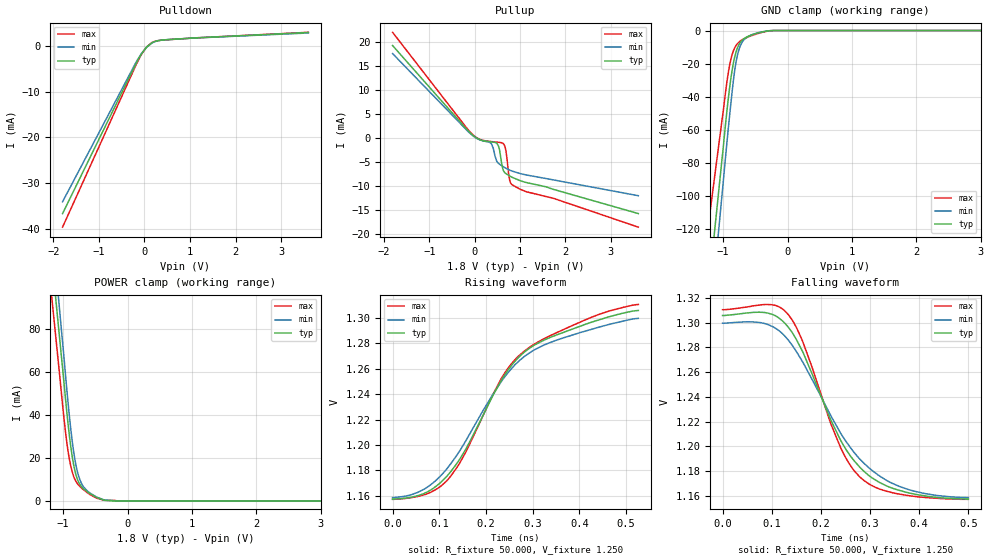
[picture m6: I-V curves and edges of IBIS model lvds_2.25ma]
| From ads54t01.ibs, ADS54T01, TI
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[Model]   lvds_2.25ma
Model_type 3-state
Vref=1.250E+00
Rref=5.000E+01
Cref=0.000E+00
Vmeas=1.250E+00
C_comp   7.860E-13   7.790E-13   7.930E-13
[Voltage Range]   1.800E+00   1.650E+00   1.950E+00
[POWER Clamp Reference]   1.800E+00   1.650E+00   1.950E+00
[GND Clamp Reference]   0.000E+00   0.000E+00   0.000E+00
[Pullup Reference]   1.800E+00   1.650E+00   1.950E+00
[Pulldown Reference]   0.000E+00   0.000E+00   0.000E+00
[Temperature Range]   25   85   -40
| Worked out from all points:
|   slope of the pulldown table from 0 to 0.27 V, typ, clamps not added: 137 ohm
|   slope of the pullup table from 0 to 0.27 V, typ, clamps not added: 279 ohm
|   GND clamp passes 1 mA (typ) near -0.41 V on its own axis
|   POWER clamp passes 1 mA (typ) near -0.41 V on its own axis
|   rising waveform, R_fixture 50.000, V_fixture 1.250: 20-80 % time 153ps typ, 161ps min, 159ps max; typ from 1.16 V to 1.31 V
|   falling waveform, R_fixture 50.000, V_fixture 1.250: 20-80 % time 107ps typ, 128ps min, 87.4ps max; typ from 1.31 V to 1.16 V
[GND Clamp]
-1.8V     -374.4mA   -423.5mA   -288.4mA
-1.02V    -78.69mA   -100.5mA   -54.92mA
-920mV    -41.17mA   -59.34mA   -25.51mA
-860mV    -23.88mA   -36.88mA   -14.48mA
-820mV    -15.94mA   -23.97mA   -10.43mA
-780mV    -10.76mA   -15.27mA   -8.038mA
-740mV    -7.589mA   -9.923mA   -6.562mA
-700mV    -5.657mA   -6.755mA   -5.499mA
-640mV    -4.069mA   -4.329mA   -4.359mA
-460mV    -1.489mA   -1.354mA   -1.806mA
-220mV    -4.201uA   -14.01uA   -11.29uA
3.6V      0A         0A         0A
[Power Clamp]
-1.8V     302.8mA    334.3mA    279.3mA
-1.76V    290.6mA    320.1mA    266.6mA
-1.06V    77.25mA    90.47mA    60.21mA
-940mV    40.5mA     50.88mA    26.54mA
-880mV    24.97mA    33.1mA     16.1mA
-820mV    14.43mA    19.78mA    10.24mA
-780mV    10.23mA    13.83mA    8.195mA
-720mV    6.913mA    8.542mA    6.262mA
-580mV    3.451mA    3.702mA    2.982mA
-360mV    441.4uA    538.8uA    356.5uA
-140mV    0A         9.789uA    18.55uA
3.6V      0A         0A         0A
[Pullup]
-1.81V    19.33mA    17.65mA    22.08mA
-30mV     540.2uA    453.4uA    652.3uA
370mV     -758.1uA   -1.136mA   -694.7uA
490mV     -1.048mA   -4.86mA    -804.7uA
530mV     -1.71mA    -5.276mA   -841.6uA
610mV     -5.976mA   -5.803mA   -982.6uA
650mV     -7.009mA   -6.039mA   -1.331mA
690mV     -7.357mA   -6.253mA   -2.621mA
770mV     -7.838mA   -6.622mA   -8.652mA
830mV     -8.153mA   -6.853mA   -9.716mA
1.15V     -9.25mA    -7.667mA   -11.17mA
3.61V     -15.7mA    -11.97mA   -18.53mA
[Pulldown]
-1.8V     -36.72mA   -34.13mA   -39.7mA
-180mV    -3.677mA   -3.428mA   -3.97mA
-80mV     -1.889mA   -1.783mA   -2.015mA
40mV      -299.8uA   -311.3uA   -270.9uA
160mV     724.9uA    669.1uA    793.7uA
320mV     1.262mA    1.247mA    1.257mA
520mV     1.453mA    1.46mA     1.421mA
3.6V      3.006mA    2.903mA    3.048mA
[Rising Waveform]
R_fixture = 50.000
V_fixture = 1.250
V_fixture_min = 1.250
V_fixture_max = 1.250
|  time   V(typ)   V(min)   V(max)
0s        1.157V     1.159V     1.157V
70ps      1.162V     1.166V     1.161V
120ps     1.177V     1.183V     1.173V
156ps     1.196V     1.203V     1.194V
234ps     1.252V     1.251V     1.253V
260ps     1.265V     1.262V     1.266V
288ps     1.275V     1.271V     1.276V
338ps     1.285V     1.281V     1.286V
428ps     1.297V     1.291V     1.301V
526ps     1.306V     1.3V       1.31V
[Falling Waveform]
R_fixture = 50.000
V_fixture = 1.250
V_fixture_min = 1.250
V_fixture_max = 1.250
|  time   V(typ)   V(min)   V(max)
0s        1.306V     1.3V       1.31V
88ps      1.308V     1.299V     1.315V
134ps     1.296V     1.286V     1.306V
164ps     1.276V     1.268V     1.284V
240ps     1.205V     1.211V     1.199V
264ps     1.19V      1.197V     1.182V
288ps     1.18V      1.186V     1.172V
334ps     1.168V     1.173V     1.164V
378ps     1.163V     1.165V     1.16V
500ps     1.157V     1.159V     1.157V
[Ramp]
dV/dt_r   8.8980E-02/1.5250E-10   8.4540E-02/1.6090E-10   9.1920E-02/1.5850E-10
dV/dt_f   8.8980E-02/1.0691E-10   8.4540E-02/1.2806E-10   9.1920E-02/8.7078E-11
R_load = 50
